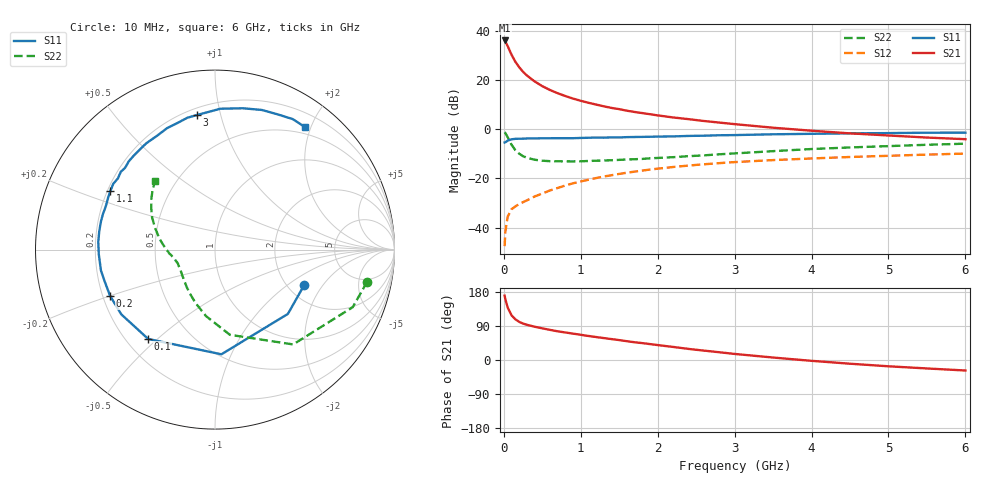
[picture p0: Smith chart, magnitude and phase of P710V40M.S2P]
! SIEMENS Small Signal Semiconductors
! BFP196
! Si NPN RF Bipolar Junction Transistor in SOT143
! VCE = 10 V  IC = 40 mA
! Common Emitter S-Parameters:  May  1996
# GHz  S  MA  R  50
!  f  S11  S21  S12  S22
! GHz  MAG  ANG  MAG  ANG  MAG  ANG  MAG  ANG
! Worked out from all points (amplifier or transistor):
!   36 points, 10 MHz to 6 GHz, reference 50 ohm
!   highest |S21| = 36.0 dB at 10 MHz (marker M1)
!   |S21| within 3 dB of that: start of sweep to 59.92 MHz
!   unconditionally stable (mu >= 1): 579.6 MHz to 4.632 GHz
!   at 250 MHz: K = 0.74, MSG = 26.5 dB, |S12| = -29.7 dB
!   at 1.4 GHz: K = 1.08, MAG = 11.9 dB, |S12| = -18.7 dB
!   at 6 GHz: K = 0.98, MSG = 2.9 dB, |S12| = -9.9 dB
!   S11 on the Smith chart (normalised r, x): 10 MHz: 2.46, -1.35; 100 MHz: 0.29, -0.47; 200 MHz: 0.23, -0.20; 1.1 GHz: 0.21, +0.25; 3 GHz: 0.24, +0.85; 6 GHz: 0.39, +1.91
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0.01  0.5351 -21.5  63.17 170.0  0.0042 73.1  0.8669 -11.9
0.02  0.5416 -41.4  59.61 160.0  0.0084 71.9  0.8316 -22.7
0.05  0.5844 -86.5  48.42 138.5  0.0167 57.0  0.6848 -50.5
0.1  0.6216 -126.8  32.43 117.9  0.0237 46.0  0.4818 -80.1
0.15  0.6347 -145.4  23.3 107.3  0.0269 44.9  0.3738 -97.7
0.2  0.6388 -156.2  18.06 100.6  0.0302 46.1  0.317 -109.9
0.25  0.6398 -164.1  14.57 96.1  0.0329 47.9  0.2818 -119.8
0.3  0.6461 -169.6  12.26 92.9  0.0358 50.0  0.2628 -126.6
0.4  0.648 -177.8  9.303 87.8  0.0428 53.1  0.2389 -137.2
0.5  0.6518 176.3  7.452 83.6  0.0492 55.0  0.2285 -144.5
0.6  0.6529 171.1  6.227 79.5  0.0569 56.7  0.2235 -149.6
0.7  0.6545 166.2  5.356 75.7  0.0638 57.6  0.2221 -153.4
0.9  0.6545 158.4  4.168 69.6  0.0794 57.6  0.2209 -159.2
1.1  0.6678 150.9  3.429 63.4  0.094 56.9  0.2255 -163.1
1.3  0.6708 143.7  2.905 57.8  0.1091 54.9  0.2306 -166.6
1.6  0.6878 134.2  2.365 49.6  0.1302 51.6  0.2419 -171.0
2.2  0.7115 117.1  1.727 34.5  0.1699 43.7  0.2693 -179.7
3  0.7567 97.5  1.263 16.0  0.2141 32.6  0.3211 167.4
3.5  0.7855 87.8  1.068 6.5  0.2351 25.9  0.3572 159.7
4.5  0.8208 71.4  0.82 -9.8  0.2718 14.4  0.4245 146.8
5.5  0.8463 59.2  0.674 -22.3  0.3037 3.9  0.4809 136.3
6  0.8472 53.7  0.625 -27.7  0.319 -1.6  0.5065 131.3
